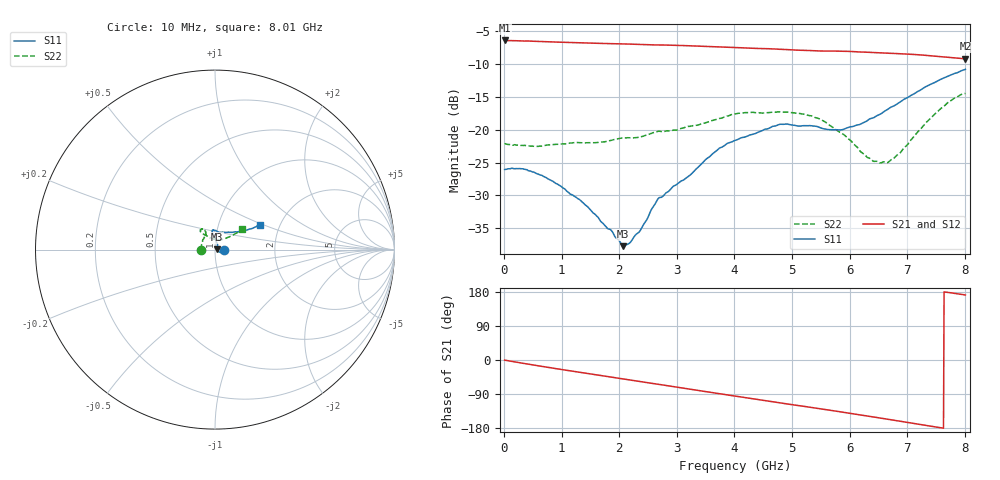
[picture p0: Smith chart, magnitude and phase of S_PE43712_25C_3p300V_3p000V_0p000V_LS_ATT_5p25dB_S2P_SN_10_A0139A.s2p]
! DEVICE ID: PE43712
! File Path: z:\PE43713\PE43713_CHAR_NOM_04292014\AMB\3p300\LS_ATT_5p25dB\PE43713_AMB_3p300V_3p000V_0p000V_LS_ATT_5p25dB_S2P_SN_10_A0139A.s2p
! Serial: 10
! Lot: A0139A
! Temp: 25C
! VDD: 3.300
! VSS: 0.000
! Control_Hi: 3.000
! Control_Lo: 0.000
! Attenuation Step: 5.25dB
! Port 1: RF1
! Port 2: RF2
! ThroughPath:1-2
! IDD: 0.0001472809
! ISS: -1.694e-007
#  Hz  S  RI  R  50
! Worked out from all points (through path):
!   801 points, 10 MHz to 8.01 GHz, reference 50 ohm
!   highest |S21| = -6.37 dB at 10 MHz (marker M1); lowest = -9.2 dB at 8.01 GHz (marker M2)
!   group delay of S21, straight-line fit = 64.7 ps
!   lowest |S11| = -37.7 dB at 2.07 GHz (marker M3), VSWR 1.03, Z = 51.3 + j0.108 ohm
!   |S11| at or under -10 dB: start of sweep to end of sweep
!   |S22| runs from -25.0 to -14.4 dB; largest |S21 - S12| = 0.0015
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1e7  0.0499 -0.000101  0.4801 -0.00274  0.4799 -0.00269  -0.0786 0.000454
3.4e8  0.0493 -0.00959  0.4698 -0.0739  0.4696 -0.0728  -0.0757 0.00638
6.3e8  0.0429 -0.0144  0.4528 -0.1312  0.4528 -0.1313  -0.0742 0.0122
9.6e8  0.0341 -0.0163  0.4251 -0.1907  0.4252 -0.1908  -0.0753 0.0196
1.35e9  0.0244 -0.0143  0.3847 -0.2523  0.3847 -0.2523  -0.0744 0.0289
1.86e9  0.0167 -0.00384  0.3204 -0.3215  0.3205 -0.3215  -0.0692 0.0461
2.07e9  0.0129 0.00105  0.2904 -0.346  0.2905 -0.3459  -0.0688 0.0526
2.18e9  0.0131 0.00414  0.274 -0.3577  0.2741 -0.3575  -0.0668 0.0558
2.36e9  0.0127 0.0113  0.2454 -0.3751  0.2454 -0.375  -0.0614 0.0633
2.68e9  0.0149 0.0261  0.1936 -0.3991  0.1937 -0.3991  -0.0527 0.0822
3.24e9  0.00653 0.0451  0.096 -0.426  0.0961 -0.4262  -0.0521 0.093
3.72e9  0.00125 0.0713  0.0121 -0.4291  0.0119 -0.429  -0.0569 0.1071
4.01e9  -0.00521 0.0829  -0.0383 -0.423  -0.0383 -0.423  -0.0671 0.1141
4.79e9  -0.0135 0.1095  -0.161 -0.3785  -0.161 -0.3787  -0.0812 0.1106
5.35e9  -0.000315 0.1072  -0.2338 -0.3266  -0.2337 -0.3264  -0.0805 0.0985
5.87e9  0.0276 0.0963  -0.293 -0.2685  -0.2925 -0.2686  -0.0499 0.079
6.39e9  0.0749 0.097  -0.3361 -0.1958  -0.3355 -0.1955  -0.00867 0.058
6.68e9  0.1076 0.0977  -0.3525 -0.1511  -0.3522 -0.1512  0.0193 0.0537
6.87e9  0.1281 0.0991  -0.3605 -0.1215  -0.3602 -0.1214  0.0364 0.0556
7.55e9  0.2075 0.1183  -0.3621 -0.0125  -0.3617 -0.0127  0.1109 0.0872
7.81e9  0.2337 0.1311  -0.3539 0.0248  -0.3536 0.0246  0.139 0.1044
8.01e9  0.2531 0.1398  -0.3442 0.0506  -0.3436 0.0501  0.1524 0.1135
